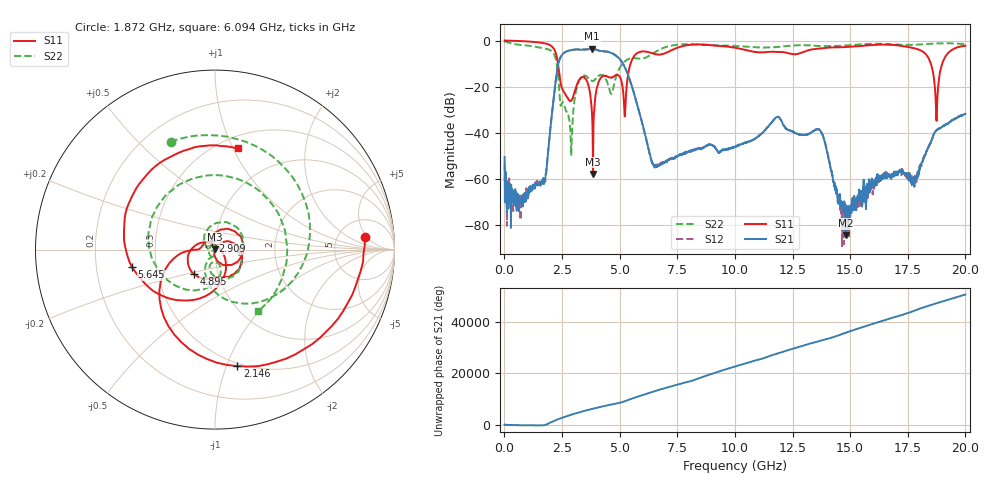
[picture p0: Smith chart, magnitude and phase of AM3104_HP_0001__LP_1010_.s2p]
!Created with skrf (http://scikit-rf.org).
# Hz S RI R 50.0
!freq ReS11 ImS11 ReS21 ImS21 ReS12 ImS12 ReS22 ImS22
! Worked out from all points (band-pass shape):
!   1601 points, 10 MHz to 20 GHz, reference 50 ohm
!   highest |S21| = -3.56 dB at 3.808 GHz (marker M1); lowest = -84.7 dB at 14.8 GHz (marker M2)
!   |S21| within 3 dB of the highest: 2.476 GHz to 4.844 GHz (2.368 GHz wide, 64.7 % of centre)
!   lowest |S11| = -57.9 dB at 3.846 GHz (marker M3), VSWR 1.00, Z = 50 + j0.124 ohm
!   |S11| at or under -10 dB: 2.324 GHz to 5.476 GHz (3.152 GHz wide, 80.8 % of centre); 18.5 GHz to 18.99 GHz (492.6 MHz wide, 2.63 % of centre)
!   |S22| runs from -50.0 to -0.2 dB; largest |S21 - S12| = 0.0046
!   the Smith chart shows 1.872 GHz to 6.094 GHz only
!   S11 on the Smith chart (normalised r, x): 1.872 GHz: 9, +4; 2.146 GHz: 0.47, -1.09; 2.909 GHz: 0.96, +0.09; 4.895 GHz: 0.77, -0.22; 5.645 GHz: 0.36, -0.09; 6.094 GHz: 0.62, +1.04
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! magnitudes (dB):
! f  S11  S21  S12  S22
! 10 MHz  0.0  -50.6  -53.9  -0.2
! 722.1 MHz  -0.2  -68.9  -72.5  -1.9
! 1.872 GHz  -1.5  -51.0  -50.8  -3.7
! 2.146 GHz  -3.6  -24.3  -24.2  -5.8
! 2.909 GHz  -26.0  -4.1  -4.1  -48.5
! 3.346 GHz  -15.9  -4.0  -4.0  -15.8
! 3.808 GHz  -33.2  -3.6  -3.5  -17.6
! 3.846 GHz  -57.9  -3.6  -3.6  -17.6
! 4.158 GHz  -16.6  -4.5  -4.5  -15.0
! 4.895 GHz  -14.9  -7.0  -7.1  -14.3
! 5.22 GHz  -33.0  -11.6  -11.6  -9.1
! 5.645 GHz  -6.5  -23.7  -23.7  -7.7
! 6.094 GHz  -4.8  -40.5  -40.5  -7.5
! 6.682 GHz  -6.1  -54.2  -54.6  -4.2
! 10.01 GHz  -3.1  -46.1  -46.6  -2.4
! 13.34 GHz  -3.8  -39.7  -39.6  -2.2
! 14.8 GHz  -2.8  -84.7  -76.2  -2.2
! 16.68 GHz  -1.8  -59.2  -58.6  -1.6
! 18.26 GHz  -5.7  -49.8  -49.4  -1.6
! 18.75 GHz  -34.9  -38.9  -38.9  -1.3
! 19.13 GHz  -7.1  -36.7  -36.6  -1.2
! 20 GHz  -2.3  -31.9  -32.0  -1.6
